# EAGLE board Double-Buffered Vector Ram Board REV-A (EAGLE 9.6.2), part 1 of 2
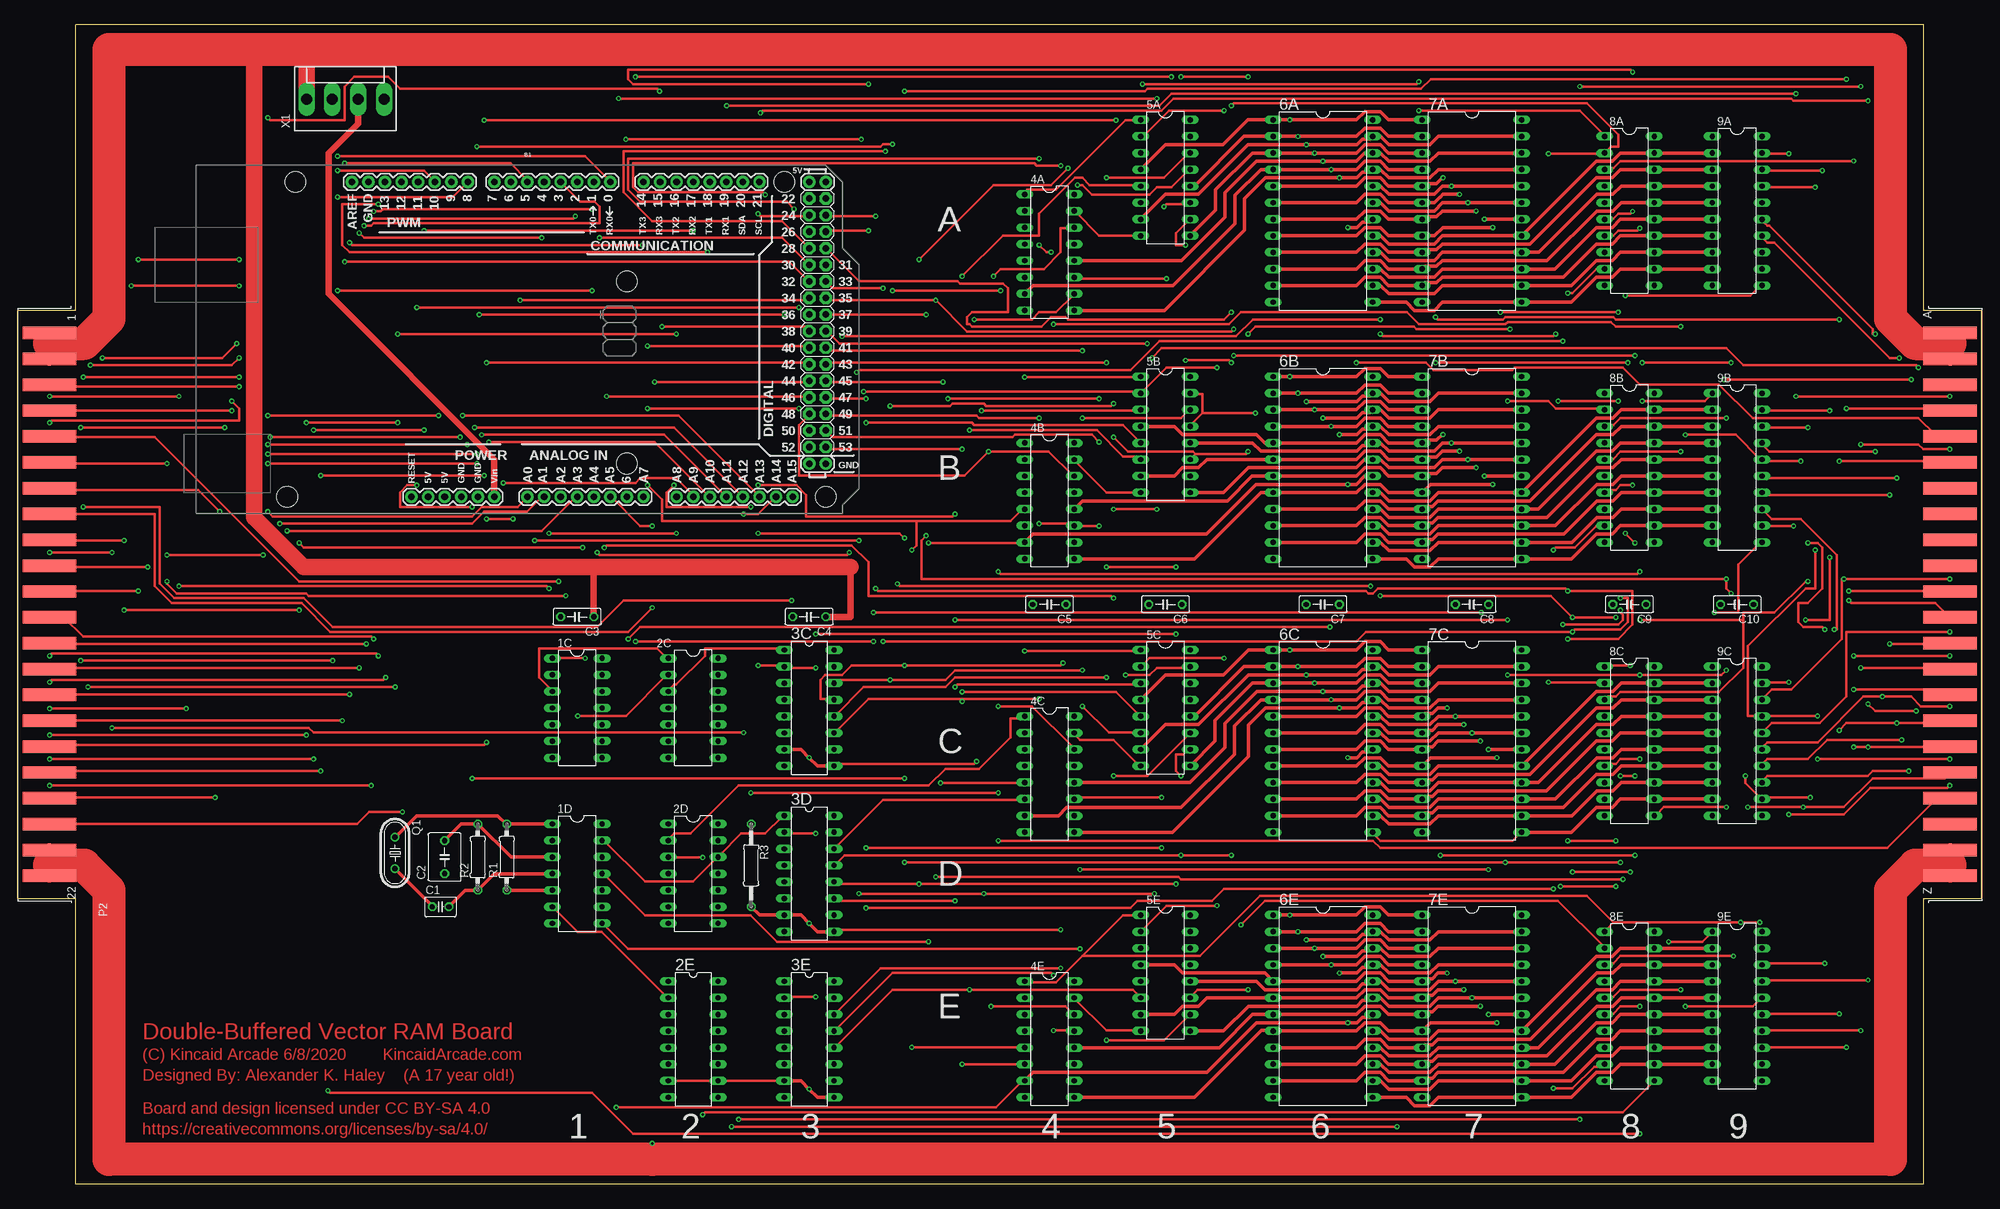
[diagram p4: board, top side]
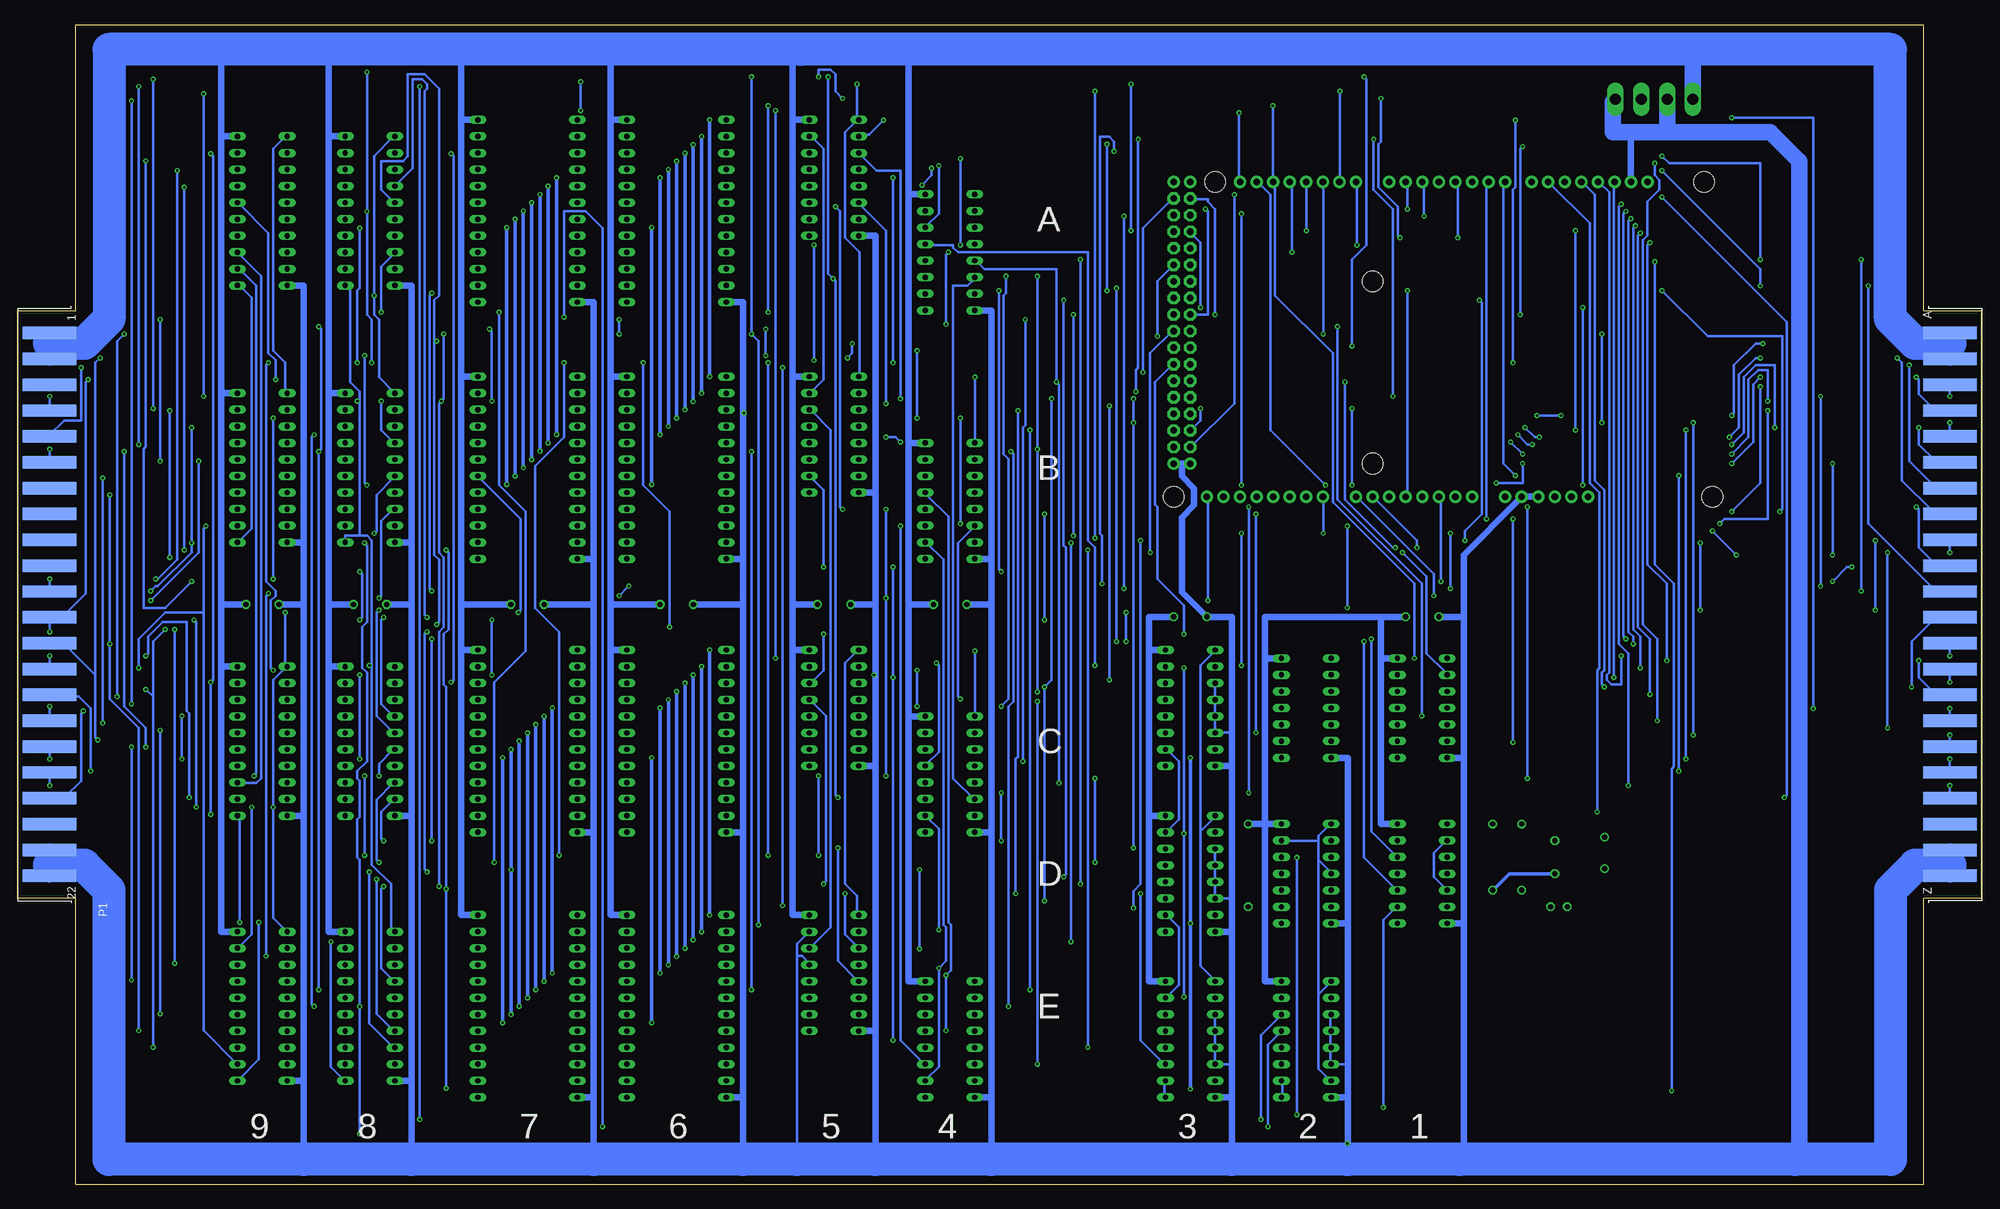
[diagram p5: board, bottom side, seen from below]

Size 300.99 x 177.8 mm. Coordinates in mm from the lower left corner, seen from the top.
Outline: 292.1,0 292.1,43.81 300.99,43.81 300.99,133.99 292.1,133.99 292.1,177.8 291.46,177.8 8.89,177.8 8.89,176.53 8.89,133.99 0,133.99 0,43.81 8.89,43.81 8.89,0 292.1,0
Copper layers (1*16): Top 0.035mm / dielectric 1.5mm / Bottom 0.035mm
Design rules "default": minimum track width 6mil, minimum drill 0.35mm, track to track 6mil, track to pad 6mil, pad to pad 6mil, via to via 6mil, smd to smd 6mil, copper to edge 40mil, drill to drill 6mil, minimum pad ring 10mil, minimum via ring 8mil, stop-mask expansion 4mil, vias tented up to drill 0mil, thermal gap 10mil
Net classes: 0 default: width 0.381 mm, clearance 0.356 mm

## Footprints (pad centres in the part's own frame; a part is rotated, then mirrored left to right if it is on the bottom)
DIL14 = drill 0.813 long: 1 -7.62,-3.81; 2 -5.08,-3.81; 3 -2.54,-3.81; 4 0,-3.81; 5 2.54,-3.81; 6 5.08,-3.81; 7 7.62,-3.81; 8 7.62,3.81; 9 5.08,3.81; 10 2.54,3.81; 11 0,3.81; 12 -2.54,3.81; 13 -5.08,3.81; 14 -7.62,3.81
DIL16 = drill 0.813 long: 1 -8.89,-3.81; 2 -6.35,-3.81; 3 -3.81,-3.81; 4 -1.27,-3.81; 5 1.27,-3.81; 6 3.81,-3.81; 7 6.35,-3.81; 8 8.89,-3.81; 9 8.89,3.81; 10 6.35,3.81; 11 3.81,3.81; 12 1.27,3.81; 13 -1.27,3.81; 14 -3.81,3.81; 15 -6.35,3.81; 16 -8.89,3.81
DIL24 = drill 0.813 long: 1 -13.97,-7.62; 2 -11.43,-7.62; 3 -8.89,-7.62; 4 -6.35,-7.62; 5 -3.81,-7.62; 6 -1.27,-7.62; 7 1.27,-7.62; 8 3.81,-7.62; 9 6.35,-7.62; 10 8.89,-7.62; 11 11.43,-7.62; 12 13.97,-7.62; 13 13.97,7.62; 14 11.43,7.62; 15 8.89,7.62; 16 6.35,7.62; 17 3.81,7.62; 18 1.27,7.62; 19 -1.27,7.62; 20 -3.81,7.62; 21 -6.35,7.62; 22 -8.89,7.62; 23 -11.43,7.62; 24 -13.97,7.62
DIL20 = drill 0.813 long: 1 -11.43,-3.81; 2 -8.89,-3.81; 3 -6.35,-3.81; 4 -3.81,-3.81; 5 -1.27,-3.81; 6 1.27,-3.81; 7 3.81,-3.81; 8 6.35,-3.81; 9 8.89,-3.81; 10 11.43,-3.81; 11 11.43,3.81; 12 8.89,3.81; 13 6.35,3.81; 14 3.81,3.81; 15 1.27,3.81; 16 -1.27,3.81; 17 -3.81,3.81; 18 -6.35,3.81; 19 -8.89,3.81; 20 -11.43,3.81
ARDUINO_MEGA = drill 1.016 pad 1.88: 0 13.97,24.13; 1 11.43,24.13; 2 8.89,24.13; 3 6.35,24.13; 3.3V -13.97,-24.13; 4 3.81,24.13; 5 1.27,24.13; 5V@0 -11.43,-24.13; 5V@1 44.45,24.13; 5V@2 46.99,24.13; 6 -1.27,24.13; 7 -3.81,24.13; 8 -7.874,24.13; 9 -10.414,24.13; 10 -12.954,24.13; 11 -15.494,24.13; 12 -18.034,24.13; 13 -20.574,24.13; 14 19.05,24.13; 15 21.59,24.13; 16 24.13,24.13; 17 26.67,24.13; 18 29.21,24.13; 19 31.75,24.13; 20 34.29,24.13; 21 36.83,24.13; A0 1.27,-24.13; A1 3.81,-24.13; A2 6.35,-24.13; A3 8.89,-24.13; A4 11.43,-24.13; A5 13.97,-24.13; A6 16.51,-24.13; A7 19.05,-24.13; A8 24.13,-24.13; A9 26.67,-24.13; A10 29.21,-24.13; A11 31.75,-24.13; A12 34.29,-24.13; A13 36.83,-24.13; A14 39.37,-24.13; A15 41.91,-24.13; AREF -25.654,24.13; GND@0 -8.89,-24.13; GND@1 -6.35,-24.13; GND@2 44.45,-19.05; GND@3 46.99,-19.05; GND@4 -23.114,24.13; RESET -16.51,-24.13; VIN -3.81,-24.13 | drill 1.016 pad 1.88 octagon: 22 44.45,21.59; 23 46.99,21.59; 24 44.45,19.05; 25 46.99,19.05; 26 44.45,16.51; 27 46.99,16.51; 28 44.45,13.97; 29 46.99,13.97; 30 44.45,11.43; 31 46.99,11.43; 32 44.45,8.89; 33 46.99,8.89; 34 44.45,6.35; 35 46.99,6.35; 36 44.45,3.81; 37 46.99,3.81; 38 44.45,1.27; 39 46.99,1.27; 40 44.45,-1.27; 41 46.99,-1.27; 42 44.45,-3.81; 43 46.99,-3.81; 44 44.45,-6.35; 45 46.99,-6.35; 46 44.45,-8.89; 47 46.99,-8.89; 48 44.45,-11.43; 49 46.99,-11.43; 50 44.45,-13.97; 51 46.99,-13.97; 52 44.45,-16.51; 53 46.99,-16.51 | hole 3.2: -34.29,24.13; -35.56,-24.13; 16.51,8.89; 16.51,-19.05; 40.64,24.13; 46.99,-24.13
C025-030X050 = drill 0.813 octagon: 1 -1.27,0; 2 1.27,0
C050-050X075 = drill 0.813 octagon: 1 -2.54,0; 2 2.54,0
C050-025X075 = drill 0.813 octagon: 1 -2.54,0; 2 2.54,0
44PINEDGE = smd 1.905 x 8.255: 1 -41.605,4.826; 2 -37.643,4.826; 3 -33.68,4.826; 4 -29.718,4.826; 5 -25.756,4.826; 6 -21.793,4.826; 7 -17.831,4.826; 8 -13.868,4.826; 9 -9.906,4.826; 10 -5.944,4.826; 11 -1.981,4.826; 12 1.981,4.826; 13 5.944,4.826; 14 9.906,4.826; 15 13.868,4.826; 16 17.831,4.826; 17 21.793,4.826; 18 25.756,4.826; 19 29.718,4.826; 20 33.68,4.826; 21 37.643,4.826; 22 41.605,4.826 | smd 1.905 x 8.255 bottom: A -41.605,4.826; B -37.643,4.826; C -33.68,4.826; D -29.718,4.826; E -25.756,4.826; F -21.793,4.826; H -17.831,4.826; J -13.868,4.826; K -9.906,4.826; L -5.944,4.826; M -1.981,4.826; N 1.981,4.826; P 5.944,4.826; R 9.906,4.826; S 13.868,4.826; T 17.831,4.826; U 21.793,4.826; V 25.756,4.826; W 29.718,4.826; X 33.68,4.826; Y 37.643,4.826; Z 41.605,4.826
HC49/S = drill 0.813: 1 -2.413,0; 2 2.413,0
0207/10 = drill 0.813 octagon: 1 -5.08,0; 2 5.08,0
0207/12 = drill 0.813 octagon: 1 -6.35,0; 2 6.35,0
KK-156-4 = drill 1.7 pad 2.184 long: 1 -5.94,0; 2 -1.98,0; 3 1.98,0; 4 5.94,0

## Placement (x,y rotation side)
1C  7432N  [DIL14]  85.72,73.03 270 top
1D  7404N  [DIL14]  85.72,47.62 270 top
2C  7400N  [DIL14]  103.5,73.03 270 top
2D  74107N  [DIL14]  103.5,47.62 270 top
2E  74161N  [DIL16]  103.5,22.23 270 top
3C  74161N  [DIL16]  121.28,73.03 270 top
3D  74161N  [DIL16]  121.28,47.62 270 top
3E  74161N  [DIL16]  121.28,22.23 270 top
4A  74157N  [DIL16]  158.12,142.88 270 top
4B  74157N  [DIL16]  158.12,104.78 270 top
4C  74157N  [DIL16]  158.12,62.87 270 top
4E  74157N  [DIL16]  158.12,22.23 270 top
5A  74157N  [DIL16]  175.9,154.31 270 top
5B  74157N  [DIL16]  175.9,114.94 270 top
5C  74157N  [DIL16]  175.9,73.03 270 top
5E  74157N  [DIL16]  175.9,32.38 270 top
6A  6116P-70  [DIL24]  200.03,149.22 270 top
6B  6116P-70  [DIL24]  200.03,109.86 270 top
6C  6116P-70  [DIL24]  200.03,67.94 270 top
6E  6116P-70  [DIL24]  200.03,27.3 270 top
7A  6116P-70  [DIL24]  222.88,149.22 270 top
7B  6116P-70  [DIL24]  222.88,109.86 270 top
7C  6116P-70  [DIL24]  222.88,67.94 270 top
7E  6116P-70  [DIL24]  222.88,27.3 270 top
8A  74HC573N  [DIL20]  247.01,149.22 270 top
8B  74HC573N  [DIL20]  247.01,109.86 270 top
8C  74HC573N  [DIL20]  247.01,67.94 270 top
8E  74HC573N  [DIL20]  247.01,27.3 270 top
9A  74HC573N  [DIL20]  263.52,149.22 270 top
9B  74HC573N  [DIL20]  263.52,109.86 270 top
9C  74HC573N  [DIL20]  263.52,67.94 270 top
9E  74HC573N  [DIL20]  263.52,27.3 270 top
B1  ARDUINO_MEGA_R3FULL  [ARDUINO_MEGA]  76.83,129.54 0 top
C1  100pf  [C025-030X050]  64.77,42.55 0 top
C2  .1uf  [C050-050X075]  65.41,50.16 90 top
C3  .1uf  [C050-025X075]  85.72,87 180 top
C4  .1uf  [C050-025X075]  121.28,87 180 top
C5  .1uf  [C050-025X075]  158.12,88.9 180 top
C6  .1uf  [C050-025X075]  175.9,88.9 180 top
C7  .1uf  [C050-025X075]  200.03,88.9 180 top
C8  .1uf  [C050-025X075]  222.88,88.9 180 top
C9  .1uf  [C050-025X075]  247.01,88.9 180 top
C10  .1uf  [C050-025X075]  263.52,88.9 180 top
P1  44PINEDGE  [44PINEDGE]  300.99,88.9 270 bottom
P2  44PINEDGE  [44PINEDGE]  0,88.9 270 top
Q1  10MHZ  [HC49/S]  57.78,50.8 270 top
R1  330  [0207/10]  74.93,50.16 90 top
R2  330  [0207/10]  70.48,50.16 90 top
R3  1K  [0207/12]  112.39,48.9 270 top
X1  [KK-156-4]  50.16,166.37 0 top

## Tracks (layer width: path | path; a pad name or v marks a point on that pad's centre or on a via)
2.5MHZ  (via drill 0.35)
  Top 0.381: v211.4,8.84 v109.39,8.84 | v217.3,132.96 217.66,132.59 227.61,132.59 227.98,132.96 244.55,132.96 244.92,132.59 v279.17,132.59 | v279.17,110.86 296.11,110.86 P1.F
  Bottom 0.381: v109.39,8.84 109.39,21.36 107.54,23.2 2E.13 | v211.4,8.84 211.4,146.58 213.98,149.16 217.3,149.16 v217.3,132.96 | v279.17,110.86 v279.17,132.59
5MHZ  (via drill 0.35)
  Top 0.381: v239.4,9.94 v110.49,9.94 | v282.49,168.31 v239.4,168.31 | v282.49,113.44 291.32,113.44 292.06,112.7 v296.11,112.7
  Bottom 0.381: v110.49,9.94 110.49,22.84 107.54,25.78 2E.14 | v239.4,168.31 v239.4,9.94 | v282.49,113.44 v282.49,168.31 | v296.11,112.7 296.11,110.86 P1.6
10MHZ
  Top 0.381: 2E.2 99.44,28.73 89.5,38.67 85.81,38.67 82.13,42.35 1D.6
+12VDC
  Top 1.016: X1.3 52.15,162.63 47.62,158.12 47.62,136.53 73.03,111.12 B1.VIN
/CS_A  (via drill 0.35)
  Top 0.381: v131.12,83.24 v94.65,83.24 | v224.29,87.66 v131.12,87.66
  Top 0.508: 7A.18 v224.79,147.96 | 7B.18 v224.79,108.58
  Bottom 0.381: v94.65,83.24 94.65,50.09 89.86,45.3 1D.10 | v131.12,87.66 v131.12,83.24 | v224.29,87.66 223.93,88.02 223.93,102.02 230.19,108.28 7B.18
  Bottom 0.508: v224.79,108.58 v224.79,147.96
/CS_B  (via drill 0.35)
  Top 0.381: v162.79,36.09 93.55,36.09 89.86,39.78 1D.8 | v225.4,48.25 v162.79,48.25
  Top 0.508: 7C.18 v225.43,66.67 | 7E.18 v225.43,26.04
  Bottom 0.381: v162.79,48.25 v162.79,36.09 | v225.4,48.25 225.43,48.25
  Bottom 0.508: v225.43,26.04 225.43,48.25 v225.43,66.67
/RESETVRAMPC
  Top 0.381: 2C.3 99.81,75.87 100.55,76.61 100.91,76.61 105.33,81.03 105.33,82.13 117.12,82.13 3C.1 | 3D.1 117.12,56.35 114.54,53.77 110.86,53.77 107.54,50.46 2D.12 107.17,50.09 103.49,46.41 96.13,46.41 89.86,52.67 1D.13
  Bottom 0.381: 119.7,54.14 119.7,33.52 117.49,31.3 3E.1 | 119.7,54.14 117.49,56.35 3D.1 | 119.7,54.14 119.7,79.55 117.49,81.76 3C.1
/TTLINVX  (via drill 0.35)
  Top 0.381: v100.55,107.17 99.44,106.07 99.44,103.86 v112.33,103.86 | v150.27,60.03 v112.33,60.03 | v150.27,52.67 207.72,52.67 208.83,51.56 286.54,51.56 293.9,58.93 296.11,58.93 P1.W
  Bottom 0.381: v100.55,107.17 109.02,115.65 109.02,151.74 110.86,153.58 B1.20 | v112.33,60.03 v112.33,103.86 | v150.27,52.67 v150.27,60.03
/TTLINVY  (via drill 0.35)
  Top 0.381: v113.81,164.26 114.17,164.63 175.31,164.63 177.15,166.47 271.81,166.47 272.17,166.1 v283.59,166.1 | v283.59,73.66 284.7,72.56 v290.96,72.56
  Bottom 0.381: v113.81,164.26 113.81,153.95 B1.21 | v283.59,73.66 v283.59,166.1 | v290.96,72.56 291.32,72.19 291.32,61.87 293.9,59.3 296.11,59.3 P1.19
/VRAMBANKSELECT  (via drill 0.35)
  Top 0.381: 163.16,34.99 169.42,41.25 172,41.25 5E.1 | 163.16,34.99 159.11,30.94 154.32,30.94 4E.1 | 2D.2 99.81,53.03 100.55,53.77 103.12,53.77 110.49,61.14 139.59,61.14 142.16,63.72 147.32,63.72 152.11,68.5 152.11,71.45 153.95,71.45 4C.1 | v154.32,81.76 172,81.76 5C.1 | 244.55,40.15 243.45,39.04 8E.1 | v267.02,40.15 v264.07,40.15 244.55,40.15 | v247.13,79.55 243.45,79.55 8C.1 | v248.97,120.07 258.55,120.07 259.65,121.17 9B.1 | 163.16,34.99 181.2,34.99 190.41,44.2 240.5,44.2 244.55,40.15
  Bottom 0.381: 5C.1 172.36,81.76 174.21,79.92 174.21,46.04 172.36,44.2 172.36,41.62 5E.1 | v154.32,81.76 154.32,71.82 4C.1 | v267.02,40.15 267.02,56.35 9C.11 | v264.07,40.15 264.07,19.15 267.02,16.2 9E.11 | 246.76,79.92 v247.13,79.55 | 246.76,79.92 246.76,98.7 247.5,99.44 248.6,99.44 | 248.6,99.44 250.81,99.44 250.81,98.7 8B.11 | 248.6,99.44 248.6,120.07 | 248.6,120.07 248.6,121.54 250.08,123.01 250.08,137.01 250.81,137.74 8A.11 | 248.6,120.07 v248.97,120.07 | 9A.1 260.02,160.58 261.86,158.74 261.86,127.8 260.02,125.96 260.02,121.54 9B.1 | 246.76,79.92 246.76,48.98 243.81,46.04 243.81,39.41 243.45,39.04 8E.1
A0_A  (via drill 0.35)
  Top 0.508: 6A.8 205.19,145.41 206.46,146.69 208.83,146.69 210.1,145.41 7A.8 217.13,145.41 218.41,146.69 v226.06,146.69 | v226.06,107.31 216.53,107.31 7B.8 210.1,106.05 208.83,107.31 206.46,107.31 205.19,106.05 6B.8 190.5,106.05 180.34,95.89 4B.9
  Bottom 0.508: v226.06,146.69 v226.06,107.31
A0_B  (via drill 0.35)
  Top 0.508: 6C.8 205.19,64.14 206.46,65.41 208.83,65.41 210.1,64.14 7C.8 216.53,65.41 v226.69,65.41 | v226.69,24.77 216.53,24.77 7E.8 210.1,23.5 208.83,24.77 206.46,24.77 205.19,23.5 6E.8 192.33,23.57 190.58,23.57 180.34,13.34 4E.9
  Bottom 0.508: v226.69,65.41 v226.69,24.77
A1_A  (via drill 0.35)
  Top 0.508: 6A.7 205.19,147.96 206.46,149.22 208.83,149.22 210.1,147.96 7A.7 215.67,148.36 217.44,148.36 218.31,149.22 v223.52,149.22 | v223.52,109.86 218.31,109.86 217.44,108.99 215.67,108.99 7B.7 210.1,108.58 208.83,109.86 206.46,109.86 205.19,108.58 6B.7 189.18,108.58 185.37,104.78 163.19,104.78 4B.12
  Bottom 0.508: v223.52,149.22 v223.52,109.86
A1_B  (via drill 0.35)
  Top 0.508: 6C.7 205.19,66.67 206.46,67.94 208.83,67.94 210.1,66.67 7C.7 215.67,67.08 216.81,67.08 217.67,67.94 v224.16,67.94 | v224.16,27.3 217.67,27.3 216.81,26.44 215.67,26.44 7E.7 210.1,26.04 208.83,27.3 206.46,27.3 205.19,26.04 6E.7 189.23,26.04 184.15,20.95 4E.12
  Bottom 0.508: v224.16,67.94 v224.16,27.3
A2_A  (via drill 0.35)
  Top 0.508: 6A.6 205.19,150.5 206.46,151.76 208.83,151.76 210.1,150.5 7A.6 217.13,150.5 218,151.36 218.03,151.36 218.44,151.76 v220.98,151.76 | v220.98,112.39 218.31,112.39 217.44,111.53 215.67,111.53 7B.6 210.1,111.12 208.83,112.39 206.46,112.39 205.19,111.12 6B.6 182.25,111.12 180.97,109.86 178.52,109.86 177.25,108.58 5B.7
  Bottom 0.508: v220.98,151.76 v220.98,112.39
A2_B  (via drill 0.35)
  Top 0.508: 6C.6 205.19,69.22 206.46,70.48 208.83,70.48 210.1,69.22 7C.6 215.67,69.62 216.81,69.62 217.67,70.48 v221.62,70.48 | v221.62,29.84 217.67,29.84 216.81,28.98 215.67,28.98 7E.6 210.1,28.57 208.83,29.84 206.46,29.84 205.19,28.57 6E.6 182.25,28.57 180.97,27.3 178.52,27.3 177.25,26.04 5E.7
  Bottom 0.508: v221.62,70.48 v221.62,29.84
A3_A  (via drill 0.35)
  Top 0.508: 6A.5 205.19,153.03 206.46,154.31 208.83,154.31 210.1,153.03 7A.5 215.67,153.44 217.44,153.44 218.31,154.31 v218.44,154.31 | v218.44,114.94 218.31,114.94 217.44,114.07 215.67,114.07 7B.5 210.1,113.67 208.83,114.94 206.46,114.94 205.19,113.67 6B.5 191.13,113.67 189.87,114.94 178.52,114.94 177.25,116.2 5B.4
  Bottom 0.508: v218.44,154.31 v218.44,114.94
A3_B  (via drill 0.35)
  Top 0.508: 6C.5 205.19,71.75 206.46,73.03 208.83,73.03 210.1,71.75 7C.5 215.67,72.16 216.81,72.16 217.67,73.03 v219.07,73.03 | v219.07,32.38 217.67,32.38 216.81,31.52 215.67,31.52 7E.5 210.1,31.11 208.83,32.38 206.46,32.38 205.19,31.11 6E.5 191.13,32.38 178.52,32.38 177.25,33.66 5E.4
  Bottom 0.508: v219.07,73.03 v219.07,32.38
A4_A  (via drill 0.35)
  Top 0.508: 7A.4 210.1,155.57 208.83,156.84 206.46,156.84 205.19,155.57 v201.29,155.57 6A.4 190.5,155.57 186.54,151.61 186.54,147.3 177.03,137.79 155.57,137.79 4A.7 | 6B.4 v201.29,116.2 205.19,116.2 206.46,117.47 208.83,117.47 210.1,116.2 7B.4
  Bottom 0.508: v201.29,155.57 v201.29,116.2
A4_B  (via drill 0.35)
  Top 0.508: 7C.4 210.1,74.3 208.83,75.56 206.46,75.56 205.19,74.3 v201.29,74.3 6C.4 190.5,74.3 186.46,70.26 186.46,65.94 178.3,57.78 160.74,57.78 159.47,56.52 4C.7 | 6E.4 v201.29,33.66 205.19,33.66 206.46,34.92 208.83,34.92 210.1,33.66 7E.4
  Bottom 0.508: v201.29,74.3 v201.29,33.66
A5_A  (via drill 0.35)
  Top 0.508: 7A.3 210.1,158.12 208.83,159.38 206.46,159.38 205.19,158.12 v198.75,158.12 6A.3 189.19,158.12 183.54,152.46 183.54,149.33 179.71,145.5 5A.9 | 6B.3 v198.75,118.75 205.19,118.75 206.46,120.02 208.83,120.02 210.1,118.75 7B.3
  Bottom 0.508: v198.75,158.12 v198.75,118.75
A5_B  (via drill 0.35)
  Top 0.508: 7C.3 210.1,76.83 208.83,78.11 206.46,78.11 205.19,76.83 v198.75,76.83 6C.3 189.23,76.83 183.51,71.12 183.51,67.94 5C.9 | 6E.3 v198.75,36.2 205.19,36.2 206.46,37.47 208.83,37.47 210.1,36.2 7E.3
  Bottom 0.508: v198.75,76.83 v198.75,36.2
A6_A  (via drill 0.35)
  Top 0.508: 7A.2 210.1,160.66 208.83,161.93 206.46,161.93 205.19,160.66 v196.22,160.66 6A.2 187.96,160.66 180.34,153.03 5A.12 | 6B.2 v196.22,121.28 205.19,121.28 206.46,122.56 208.83,122.56 210.1,121.28 7B.2
  Bottom 0.508: v196.22,160.66 v196.22,121.28
A6_B  (via drill 0.35)
  Top 0.508: 7C.2 210.1,79.38 208.83,80.64 206.46,80.64 205.19,79.38 v196.22,79.38 6C.2 187.96,79.38 180.34,71.75 5C.12 | 6E.2 v196.22,38.73 205.19,38.73 206.46,40.01 208.83,40.01 210.1,38.73 7E.2
  Bottom 0.508: v196.22,79.38 v196.22,38.73
A7_A  (via drill 0.35)
  Top 0.508: 7A.1 210.1,163.19 208.83,164.47 206.46,164.47 205.19,163.19 v194.94,163.19 6A.1 188.51,163.19 184.7,159.38 175.9,159.38 5A.4 | 6B.1 v194.94,123.83 205.19,123.83 206.46,125.09 208.83,125.09 210.1,123.83 7B.1
  Bottom 0.508: v194.94,123.83 v194.94,163.19
A7_B  (via drill 0.35)
  Top 0.508: 7C.1 210.1,81.92 208.83,83.19 206.46,83.19 205.19,81.92 v194.94,81.92 6C.1 188.59,81.92 184.78,78.11 175.9,78.11 5C.4 | 6E.1 v194.94,41.27 205.19,41.27 206.46,42.55 208.83,42.55 210.1,41.27 7E.1
  Bottom 0.508: v194.94,41.27 v194.94,81.92
A8_A  (via drill 0.35)
  Top 0.508: 7B.23 217.72,121.28 216.45,120.02 210.15,120.02 208.88,121.28 6B.23 207.24,120.88 206.1,120.88 205.24,120.02 v197.49,120.02 | 7A.23 217.72,160.66 216.45,159.38 210.15,159.38 208.88,160.66 6A.23 207.24,160.25 206.1,160.25 205.24,159.38 v197.49,159.38 188.56,159.38 180.94,151.76 175.9,151.76 5A.7
  Bottom 0.508: v197.49,120.02 v197.49,159.38
A8_B  (via drill 0.35)
  Top 0.508: 7C.23 217.72,79.38 216.45,78.11 210.15,78.11 208.88,79.38 6C.23 207.24,78.97 206.1,78.97 205.24,78.11 v197.49,78.11 188.59,78.11 180.97,70.48 175.9,70.48 5C.7 | 7E.23 217.72,38.73 216.45,37.47 210.15,37.47 208.88,38.73 6E.23 207.24,38.33 206.1,38.33 205.24,37.47 v197.49,37.47
  Bottom 0.508: v197.49,37.47 v197.49,78.11
A9_A  (via drill 0.35)
  Top 0.508: 7B.22 217.72,118.75 216.45,117.47 210.15,117.47 208.88,118.75 6B.22 207.24,118.34 206.1,118.34 205.24,117.47 v200.03,117.47 | 7A.22 217.72,158.12 216.45,156.84 210.15,156.84 208.88,158.12 6A.22 206.41,158.12 205.14,156.84 v200.03,156.84 189.87,156.84 185.04,152.02 185.04,148.29 178.35,141.6 4A.12
  Bottom 0.508: v200.03,117.47 v200.03,156.84
A9_B  (via drill 0.35)
  Top 0.508: 7C.22 217.72,76.83 216.45,75.56 210.15,75.56 208.88,76.83 6C.22 207.24,76.43 206.1,76.43 205.24,75.56 v200.03,75.56 189.95,75.56 185.01,70.63 185.01,66.99 179.62,61.59 4C.12 | 7E.22 217.72,36.2 216.45,34.92 210.15,34.92 208.88,36.2 6E.22 207.24,35.79 206.1,35.79 205.24,34.92 v200.03,34.92
  Bottom 0.508: v200.03,34.92 v200.03,75.56
A10_A  (via drill 0.35)
  Top 0.508: 7B.19 v222.25,111.12 218.36,111.12 217.09,109.86 210.15,109.86 208.88,111.12 6B.19 206.41,111.12 205.14,109.86 188.59,109.86 184.78,106.05 5B.9 | 6A.19 208.88,150.5 210.15,149.22 217.09,149.22 218.36,150.5 v222.25,150.5 7A.19
  Bottom 0.508: v222.25,111.12 v222.25,150.5
A10_B  (via drill 0.35)
  Top 0.508: 6C.19 208.88,69.22 210.15,67.94 216.45,67.94 217.72,69.22 v222.88,69.22 7C.19 | 7E.19 v222.88,28.57 217.72,28.57 216.45,27.3 210.15,27.3 208.88,28.57 6E.19 207.24,28.17 206.1,28.17 205.24,27.3 188.59,27.3 184.78,23.5 5E.9
  Bottom 0.508: v222.88,28.57 v222.88,69.22
CS_A  (via drill 0.35)
  Top 0.381: v139.59,37.2 116.38,37.2 112.33,41.25 96.13,41.25 89.86,47.51 1D.11 | v139.59,98.34 153.95,98.34 4B.7
  Top 0.508: 6B.18 206.41,108.58 205.14,107.31 v203.84,107.31 189.77,107.31 182.15,99.69 155.57,99.69 4B.7 | 6A.18 207.24,147.55 206.1,147.55 205.24,146.69 v203.84,146.69
  Bottom 0.381: v139.59,98.34 v139.59,37.2
  Bottom 0.508: v203.84,146.69 v203.84,107.31
CS_B  (via drill 0.35)
  Top 0.381: v91.71,11.79 149.9,11.79 153.95,15.84 4E.7
  Top 0.508: 6C.18 207.24,66.27 206.1,66.27 205.24,65.41 v203.84,65.41 | 6E.18 207.24,25.63 206.1,25.63 205.24,24.77 v203.84,24.77 189.87,24.77 182.25,17.14 155.57,17.14 4E.7
  Bottom 0.381: v91.71,11.79 91.71,40.51 89.86,42.35 1D.9
  Bottom 0.508: v203.84,65.41 v203.84,24.77
CSIN  (via drill 0.35)
  Top 0.381: v137.01,20.99 153.95,20.99 4E.5 | v137.01,97.23 137.74,97.97 137.74,101.65 | 137.74,101.65 152.11,101.65 153.95,103.49 4B.5 | v96.5,118.96 v119.7,118.96 | v96.5,107.17 98.7,104.97 98.7,101.65 137.74,101.65
  Bottom 0.381: v137.01,97.23 v137.01,20.99 | v119.7,118.96 119.7,117.12 121.17,115.65 B1.50 | v96.5,107.17 v96.5,118.96
D0  (via drill 0.35)
  Top 0.381: v48.98,157.63 86.92,157.63 90.6,153.95 B1.0 | v18.47,90.97 4.84,90.97 P2.11 | v18.47,141.8 v33.88,141.8
  Bottom 0.381: v48.98,157.63 47.88,156.53 33.88,156.53 v33.88,141.8 | v18.47,90.97 v18.47,141.8
D1  (via drill 0.35)
  Top 0.381: v88.02,149.53 55.98,149.53 55.61,149.16 v54.51,149.16 | v54.51,83.6 54.14,83.97 9.99,83.97 7.05,86.92 P2.12
  Bottom 0.381: v88.02,149.53 88.02,153.58 B1.1 | v54.51,149.16 54.88,148.79 54.88,83.97 v54.51,83.6
D2  (via drill 0.35)
  Top 0.381: v85.45,148.43 85.08,148.06 v53.77,148.06 | v53.4,82.87 4.84,82.87 P2.13
  Bottom 0.381: v85.45,148.43 85.45,153.58 B1.2 | v53.77,148.06 54.14,147.69 54.14,84.71 53.4,83.97 v53.4,82.87
D3  (via drill 0.35)
  Top 0.381: v53.03,146.95 54.14,146.95 54.51,147.32 89.13,147.32 89.13,149.9 88.39,150.63 86.18,150.63 83.24,153.58 B1.3 | v52.3,79.18 4.84,79.18 P2.14
  Bottom 0.381: v53.03,146.95 53.4,146.58 53.4,85.08 52.3,83.97 v52.3,79.18
D4  (via drill 0.35)
  Top 0.381: v80.29,145.11 53.03,145.11 v52.3,145.85 | v50.83,75.13 4.84,75.13 P2.15
  Bottom 0.381: v80.29,145.11 80.29,153.58 B1.4 | v52.3,145.85 52.67,145.48 52.67,85.45 50.83,83.6 v50.83,75.13
D5  (via drill 0.35)
  Top 0.381: v50.09,156.53 75.5,156.53 78.08,153.95 B1.5 | v49.72,71.08 4.84,71.08 P2.16
  Bottom 0.381: v50.09,156.53 50.09,154.69 49.35,153.95 49.35,152.48 51.19,150.63 51.19,145.48 51.93,144.74 51.93,85.81 49.72,83.6 v49.72,71.08
D6  (via drill 0.35)
  Top 0.381: v71.82,102.02 v75.87,102.02 | v71.82,67.77 71.45,67.4 4.84,67.4 P2.17
  Bottom 0.381: v75.87,102.02 75.87,153.58 B1.6 | v71.82,67.77 v71.82,102.02
D7  (via drill 0.35)
  Top 0.381: v46.41,108.65 v71.45,108.65 | v46.41,63.35 4.84,63.35 P2.18
  Bottom 0.381: v71.45,108.65 73.29,110.49 73.29,153.58 B1.7 | v46.41,63.35 v46.41,108.65
D8  (via drill 0.35)
  Top 0.381: B1.8 66.66,151.37 v48.98,151.37 | v30.2,59.3 4.84,59.3 P2.19
  Bottom 0.381: v48.98,151.37 29.83,132.22 29.83,59.66 v30.2,59.3
D9  (via drill 0.35)
  Top 0.381: v58.93,57.09 53.85,57.09 52.01,55.24 4.84,55.24 P2.20
  Bottom 0.381: v58.93,57.09 58.93,78.82 58.56,79.18 58.56,106.07 60.03,107.54 60.03,147.32 66.29,153.58 B1.9
D10  (via drill 0.35)
  Top 0.381: v48.98,155.42 62.24,155.42 63.72,153.95 B1.10 | v33.88,137.74 v17.36,137.74
  Bottom 0.381: v48.98,155.42 33.88,140.32 v33.88,137.74 | v17.36,137.74 17.36,101.28 7.05,90.97 4.84,90.97 P2.M
D11  (via drill 0.35)
  Top 0.381: v57.82,76.24 v10.73,76.24
  Bottom 0.381: v57.82,76.24 58.19,76.61 58.19,78.45 57.82,78.82 57.82,106.44 59.3,107.91 59.3,151.74 61.14,153.58 B1.11 | v10.73,76.24 10.73,83.24 7.05,86.92 P2.N
D12  (via drill 0.35)
  Top 0.381: v55.24,81.03 54.88,81.39 5.21,81.39 v4.84,81.03
  Bottom 0.381: v55.24,81.03 55.24,76.61 56.72,76.61 57.45,77.34 57.45,78.08 57.09,78.45 57.09,152.11 58.56,153.58 B1.12 | v4.84,81.03 4.84,82.87 P2.P
D13  (via drill 0.35)
  Top 0.381: v56.35,77.71 55.98,77.34 5.21,77.34 v4.84,76.97
  Bottom 0.381: v56.35,77.71 56.35,153.58 B1.13 | v4.84,76.97 4.84,78.82 P2.R
D14  (via drill 0.35)
  Top 0.381: v95.76,144 51.19,144 v50.83,144.37 | v9.63,80.29 v48.25,80.29
  Bottom 0.381: v95.76,144 95.76,153.58 B1.14 | v50.83,144.37 51.19,144 51.19,95.02 48.25,92.08 v48.25,80.29 | v9.63,80.29 9.63,77.71 7.05,75.13 4.84,75.13 P2.S
D15  (via drill 0.35)
  Top 0.381: v98.34,167.58 97.97,167.94 58.56,167.94 56.72,169.79 51.56,169.79 50.09,168.31 50.09,163.16 38.67,163.16 v38.3,163.53 | v4.84,72.92 v25.78,72.92
  Bottom 0.381: v98.34,167.58 98.34,153.95 B1.15 | v38.3,163.53 25.78,163.53 v25.78,72.92 | v4.84,72.92 4.84,71.08 P2.T
D16  (via drill 0.35)
  Top 0.381: v58.19,130.38 v100.91,130.38 | v44.2,116.75 v58.19,116.75 | v44.2,68.87 v4.84,68.87
  Bottom 0.381: v100.91,130.38 100.91,153.58 B1.16 | v58.19,116.75 v58.19,130.38 | v44.2,68.87 v44.2,116.75 | v4.84,68.87 4.84,67.4 P2.U
D17  (via drill 0.35)
  Top 0.381: v62.24,146.22 v103.49,146.22 | v45.3,115.65 v62.24,115.65 | v4.84,65.19 v45.3,65.19
  Bottom 0.381: v103.49,146.22 103.49,153.58 B1.17 | v62.24,115.65 v62.24,146.22 | v45.3,65.19 v45.3,115.65 | v4.84,65.19 4.84,63.35 P2.V
D18  (via drill 0.35)
  Top 0.381: v105.7,142.9 50.83,142.9 49.72,144 49.72,150.27 v55.24,150.27 | v54.14,61.14 v4.84,61.14
  Bottom 0.381: v105.7,142.9 105.7,153.58 B1.18 | v55.24,150.27 55.61,149.9 55.61,82.87 54.14,81.39 v54.14,61.14 | v4.84,61.14 4.84,59.3 P2.W
FRAMECOMPLETE  (via drill 0.35)
  Top 0.381: v86.92,80.66 82.13,80.66 1C.1 | v272.54,120.8 v296.11,120.8 | v272.54,167.21 176.78,167.21 174.94,165.37 v108.65,165.37
  Bottom 0.381: v86.92,80.66 86.92,92.08 99.44,104.6 99.44,127.43 108.28,136.27 108.28,153.58 B1.19 108.65,153.95 v108.65,165.37 | v296.11,120.8 296.11,118.96 P1.4 | v272.54,167.21 v272.54,120.8
GND  (via drill 0.35)
  Top 0.381: 181.57,118.22 179.73,116.38 5B.13 | 181.57,118.22 181.57,121.17 179.73,121.17 5B.15 | 4E.15 162.05,28.36 166.84,23.57 172,23.57 5E.8 | 4C.15 162.05,68.87 162.79,68.14 167.94,68.14 171.63,64.45 172,64.45 5C.8 | 4B.15 162.05,110.86 166.84,106.07 172,106.07 5B.8 | 4A.15 162.05,149.16 165.74,145.48 172,145.48 5A.8 | v169.79,78.08 173.47,78.08 174.57,79.18 179.36,79.18 5C.15 | v189.67,118.22 181.57,118.22 | v97.23,6.26 97.23,3.81
  Top 2.032: P2.22 4.83,48.9 P2.21 | P1.Z 296.16,48.9 P1.Y
  Top 5.08: 4.83,48.9 10.16,48.9 13.97,45.09 13.97,3.81 97.23,3.81 287.02,3.81 287.02,45.09 290.83,48.9 296.16,48.9
  Bottom 0.381: 5A.15 179.36,160.58 177.52,158.74 177.52,123.38 179.36,121.54 5B.15 | 3C.3 117.49,76.61 117.49,74.4 3C.4 117.49,74.03 117.49,71.82 3C.5 117.49,71.45 117.49,69.24 3C.6 117.12,69.24 114.94,69.24 | 3D.3 117.49,51.19 117.49,48.98 3D.4 117.49,48.62 117.49,46.41 3D.5 117.49,46.04 117.49,43.83 3D.6 117.12,43.83 114.94,43.83 | 3E.3 117.49,25.78 117.49,23.57 3E.4 117.49,23.2 117.49,20.99 3E.5 117.49,20.62 117.49,18.41 3E.6 114.94,18.41 | 2E.3 99.81,25.78 99.81,23.57 2E.4 99.81,23.2 99.81,20.99 2E.5 99.81,20.62 99.81,18.41 2E.6 97.16,18.41 | 181.57,34.99 180.84,34.99 179.73,33.88 5E.13 | 181.57,34.99 181.57,36.83 179.73,38.67 5E.15 | v169.79,78.08 169.54,78.08 | 181.57,3.81 181.57,34.99 | v189.67,118.22 189.87,118.22 | v97.23,6.26 97.23,3.81
  Bottom 1.016: 4E.8 151.76,13.34 | 151.76,13.34 151.76,3.81 | 6E.12 189.87,13.34 | 189.87,3.81 189.87,13.34 | 5E.8 169.54,23.5 | 169.54,3.81 169.54,23.5 | 7E.12 212.72,13.34 | 212.72,3.81 212.72,13.34 | 8E.10 240.66,15.88 | 240.66,3.81 240.66,15.88 | 9E.10 257.18,15.88 | 257.18,15.88 257.18,3.81 | 257.18,15.88 257.18,56.52 | 257.18,56.52 257.18,88.9 | 257.18,88.9 257.18,98.42 | 257.18,98.42 257.18,137.79 9A.10 | 257.18,98.42 9B.10 | 257.18,88.9 C10.2 | 257.18,56.52 9C.10 | 240.66,15.88 240.66,56.52 | 240.66,56.52 240.66,88.9 | 240.66,88.9 240.66,98.42 | 240.66,98.42 240.66,137.79 8A.10 | 240.66,98.42 8B.10 | 8C.10 240.66,56.52 | 212.72,13.34 212.72,53.98 | 212.72,53.98 212.72,88.9 | 212.72,88.9 212.72,95.89 | 212.72,95.89 212.72,135.25 7A.12 | 212.72,95.89 7B.12 | 212.72,53.98 7C.12 | 189.87,13.34 189.87,53.98 | 189.87,53.98 189.87,88.9 | 189.87,88.9 189.87,95.89 | 189.87,95.89 189.87,118.22 189.87,135.25 6A.12 | 189.87,95.89 6B.12 | 189.87,53.98 6C.12 | 169.54,23.5 169.54,64.14 | 169.54,64.14 169.54,78.08 169.54,88.9 | 169.54,88.9 169.54,106.05 | 169.54,106.05 169.54,145.41 5A.8 | 169.54,106.05 5B.8 | 169.54,64.14 5C.8 | 151.76,13.34 151.76,53.98 | 151.76,53.98 151.76,88.9 | 151.76,88.9 151.76,95.89 | 151.76,95.89 151.76,133.99 4A.8 | 151.76,95.89 4B.8 | 151.76,53.98 4C.8 | 240.66,88.9 C9.2 | C8.2 212.72,88.9 | C7.2 189.87,88.9 | C6.2 169.54,88.9 | C5.2 151.76,88.9 | 3E.8 114.94,13.34 | 114.94,13.34 114.94,3.81 | 114.94,13.34 114.94,18.41 114.94,38.73 | 114.94,38.73 114.94,43.83 114.94,64.14 | 3C.8 114.94,64.14 | 114.94,38.73 3D.8 | 2E.8 97.16,13.34 | 97.16,13.34 97.16,3.81 | 97.16,13.34 97.16,18.41 97.16,40.01 | 97.16,40.01 97.16,65.41 2C.7 | 2D.7 97.16,40.01 | 114.94,64.14 114.94,69.24 114.94,87 C4.2 122.56,90.81 122.56,102.26 120.7,104.12 120.7,106.7 122.56,108.56 122.56,110.49
  Bottom 1.016: 1D.7 79.38,40.01 | 79.38,40.01 79.38,4.45 80.01,3.81 | 79.38,40.01 79.38,65.41 | 79.38,65.41 1C.7 | 79.38,65.41 79.38,87 | 79.38,87 C3.2 | B1.GND@4 53.72,161.04 53.98,161.29 | 122.56,110.49 B1.GND@2 | 122.56,110.49 B1.GND@3 | B1.GND@0 B1.GND@1 71.22,104.67 71.22,104.66 79.38,96.51 79.38,87
  Bottom 2.032: P2.22 4.83,48.9 P2.21 | P1.Z 296.16,48.9 P1.Y
  Bottom 2.54: X1.2 48.19,161.37 48.26,161.29 | 48.26,161.29 53.98,161.29 56.52,161.29 56.52,165.96 X1.4 | 48.26,161.29 32.38,161.29 27.94,156.84 27.94,4.45 28.57,3.81
  Bottom 5.08: 4.83,48.9 10.16,48.9 13.97,45.09 13.97,3.81 28.57,3.81 80.01,3.81 97.16,3.81 97.23,3.81 114.94,3.81 151.76,3.81 169.54,3.81 181.57,3.81 189.87,3.81 212.72,3.81 240.66,3.81 257.18,3.81 287.02,3.81 287.02,45.09 290.83,48.9 296.16,48.9
N$2
  Top 0.381: 1C.3 81.76,75.87 79.92,77.71 79.92,82.13 97.97,82.13 99.44,80.66 2C.1
N$5
  Bottom 0.381: 3D.15 124.85,54.14 123.01,55.98 123.01,64.82 124.85,66.66 3C.10
N$6
  Bottom 0.381: 3E.15 124.85,28.73 123.01,30.57 123.01,39.41 124.85,41.25 3D.10
N$48
  Top 0.508: 1D.1 R1.2 74.82,55.24 73.55,56.52 61.09,56.52 Q1.1
N$52
  Top 0.508: 1D.5 R1.1
  Bottom 0.381: 1D.5 83.97,47.14 83.97,50.83 82.13,52.67 1D.2
  Bottom 0.508: C2.1 72.39,47.62 R1.1
N$61
  Top 0.508: 1D.3 75.56,50.16 R2.2 67.94,55.24 C2.2
N$69
  Top 0.508: Q1.2 63.5,42.67 C1.1
N$74
  Top 0.508: 1D.4 73.03,47.62 R2.1 68.58,45.09 C1.2
OE_A  (via drill 0.35)
  Top 0.508: 7B.20 v219.71,113.67 218.36,113.67 217.09,112.39 210.15,112.39 208.88,113.67 6B.20 207.24,113.26 206.1,113.26 205.24,112.39 190.5,112.39 189.23,113.67 5B.12 | 6A.20 208.88,153.03 210.15,151.76 217.09,151.76 218.36,153.03 v219.71,153.03 7A.20
  Bottom 0.508: v219.71,113.67 v219.71,153.03
OE_B  (via drill 0.35)
  Top 0.508: 6C.20 208.88,71.75 210.15,70.48 216.45,70.48 217.72,71.75 v220.34,71.75 7C.20 | 7E.20 v220.34,31.11 217.72,31.11 216.45,29.84 210.15,29.84 208.88,31.11 6E.20 207.24,30.71 206.1,30.71 205.24,29.84 191.13,29.84 189.87,31.11 5E.12
  Bottom 0.508: v220.34,31.11 v220.34,71.75
OEIN  (via drill 0.35)
  Top 0.381: v163.16,127.8 124.48,127.8 124.12,128.17 B1.41 | v163.16,117.49 178.26,117.49 179.36,118.59 5B.14
  Bottom 0.381: 5E.14 179.36,36.46 176.42,39.41 176.42,115.65 179.36,118.59 5B.14 | v163.16,117.49 v163.16,127.8
P  (via drill 0.35)
  Top 0.381: 2E.7 99.81,15.84 107.17,15.84 2E.10 107.54,15.84 117.12,15.84 3E.7 | v159.84,39.04 125.22,39.04 3D.9 | v146.58,132.59 155.42,132.59 156.53,133.69 159.11,133.69 161.68,136.27 4A.10 | v146.95,64.82 146.58,64.45 125.22,64.45 3C.9
  Top 0.508: R3.2 113.67,41.27 3D.7 120.02,41.27 v121.28,40.01 122.56,38.73 3D.9 | 3C.9 122.56,64.14 v121.28,65.41 120.02,66.67 3C.7 | 3E.9 122.56,13.34 v121.28,14.61 120.02,15.88 3E.7
  Bottom 0.381: 101.65,49.72 99.81,47.88 2D.4 | 101.65,52.67 101.65,53.4 99.81,55.24 2D.1 | 101.65,52.67 101.65,49.72 | 101.65,52.67 107.17,52.67 2D.13 | 2E.9 107.17,13.63 107.17,15.84 2E.10 | 101.65,29.1 99.81,30.94 2E.1 | 101.65,29.1 101.65,17.68 99.81,15.84 2E.7 | 101.65,29.1 101.65,49.72 | 3E.10 125.22,15.84 125.22,13.63 3E.9 | v159.84,39.04 159.84,54.51 161.68,56.35 4C.10 | v146.58,132.59 146.58,116.38 146.95,116.01 v146.95,64.82
  Bottom 0.508: v121.28,14.61 v121.28,40.01 v121.28,65.41
PORTF0  (via drill 0.35)
  Top 0.381: v38.3,103.12 39.04,102.39 69.61,102.39 71.08,103.86 76.61,103.86 78.08,105.33 B1.A0 | v33.88,122.28 4.84,122.28 P2.3
  Bottom 0.381: v38.3,103.12 33.88,107.54 v33.88,122.28
PORTF1  (via drill 0.35)
  Top 0.381: v40.15,101.28 69.61,101.28 71.45,103.12 78.08,103.12 80.29,105.33 B1.A1 | v32.78,118.59 4.84,118.59 P2.4
  Bottom 0.381: v40.15,101.28 39.41,102.02 32.78,102.02 v32.78,118.59
PORTF2  (via drill 0.35)
  Top 0.381: v82.87,92.44 43.09,92.44 20.99,114.54 4.84,114.54 P2.5
  Bottom 0.381: v82.87,92.44 82.87,105.33 B1.A2
PORTF3  (via drill 0.35)
  Top 0.381: v41.25,100.18 80.29,100.18 85.45,105.33 B1.A3 | v22.84,96.5 v37.57,96.5 | v22.84,110.49 4.84,110.49 P2.6
  Bottom 0.381: v37.57,96.5 v41.25,100.18 | v22.84,110.49 v22.84,96.5
PORTF4  (via drill 0.35)
  Top 0.381: v48.98,137.01 v88.02,137.01 | v30.94,103.12 27.62,106.44 4.84,106.44 P2.7
  Bottom 0.381: v88.02,137.01 88.02,105.7 B1.A4 | v48.98,137.01 41.99,130.01 30.57,130.01 30.57,103.49 v30.94,103.12
PORTF5  (via drill 0.35)
  Top 0.381: v97.23,100.91 95.39,100.91 90.97,105.33 B1.A5 | v97.23,88.39 93.55,84.71 47.88,84.71 43.46,89.13 23.57,89.13 20.99,91.71 20.99,102.76 4.84,102.76 P2.8
  Bottom 0.381: v97.23,88.39 v97.23,100.91
PORTF6  (via drill 0.35)
  Top 0.381: v86.55,97.6 43.83,97.6 v43.09,98.34 | v16.26,98.7 4.84,98.7 P2.9 | v16.26,88.02 v43.09,88.02
  Bottom 0.381: v86.55,97.6 86.55,98.7 93.18,105.33 B1.A6 | v43.09,88.02 v43.09,98.34 | v16.26,98.7 v16.26,88.02
PORTF7  (via drill 0.35)
  Top 0.381: v83.97,90.23 44.56,90.23 44.2,90.6 24.31,90.6 22.84,92.08 v22.84,92.44 | v19.89,94.65 4.84,94.65 P2.10
  Bottom 0.381: v83.97,90.23 83.97,93.55 95.76,105.33 B1.A7 | v22.84,92.44 20.62,94.65 v19.89,94.65
PORTK0  (via drill 0.35)
  Top 0.381: v81.39,99.81 v100.91,99.81 | v81.39,91.34 81.03,91.71 v24.68,91.71 | v24.68,120.8 v4.84,120.8
  Bottom 0.381: v100.91,99.81 100.91,105.33 B1.A8 | v81.39,91.34 v81.39,99.81 | v24.68,120.8 v24.68,91.71 | v4.84,120.8 4.84,122.28 P2.C
PORTK1  (via drill 0.35)
  Top 0.381: v74.4,107.54 94.65,107.54 95.39,108.28 100.91,108.28 103.49,105.7 B1.A9 | v38.3,110.49 v70.34,110.49 | v9.99,123.75 v33.88,123.75
  Bottom 0.381: v74.4,107.54 70.34,107.54 v70.34,110.49 | v38.3,110.49 34.99,113.81 34.99,122.64 v33.88,123.75 | v9.99,123.75 9.63,123.38 9.63,121.17 7.42,118.96 4.84,118.96 P2.D
PORTK2  (via drill 0.35)
  Top 0.381: v72.19,113.81 97.6,113.81 105.7,105.7 B1.A10 | v38.3,111.96 v70.34,111.96 | v32.78,120.07 33.88,118.96 33.88,117.12 5.21,117.12 v4.84,116.75
  Bottom 0.381: v70.34,111.96 v72.19,113.81 | v38.3,111.96 35.73,114.54 35.73,123.38 34.25,124.85 32.78,124.85 v32.78,120.07 | v4.84,116.75 4.84,114.91 P2.E
PORTK3  (via drill 0.35)
  Top 0.381: v71.08,114.91 99.07,114.91 108.28,105.7 B1.A11 | v38.3,113.44 v68.87,113.44 | v9.63,116.01 v31.67,116.01
  Bottom 0.381: v71.08,114.91 69.61,113.44 v68.87,113.44 | v38.3,113.44 36.46,115.28 36.46,123.75 34.62,125.59 31.67,125.59 v31.67,116.01 | v9.63,116.01 9.63,113.44 7.05,110.86 4.84,110.86 P2.F
PORTK4  (via drill 0.35)
  Top 0.381: v69.98,116.01 100.55,116.01 110.86,105.7 B1.A12 | v38.67,114.54 v67.77,114.54 | v33.88,126.69 32.78,125.59 v11.1,125.59
  Bottom 0.381: v69.98,116.01 68.5,114.54 v67.77,114.54 | v38.67,114.54 37.2,116.01 37.2,124.12 34.62,126.69 v33.88,126.69 | v11.1,125.59 11.1,110.86 7.05,106.81 4.84,106.81 P2.H
PORTK5  (via drill 0.35)
  Top 0.381: v68.14,117.86 101.28,117.86 113.44,105.7 B1.A13 | v38.3,117.86 v64.45,117.86 | v33.52,128.91 31.3,126.69 v12.94,126.69
  Bottom 0.381: v64.45,117.86 v68.14,117.86 | v38.3,117.86 37.94,118.22 37.94,125.59 34.62,128.91 v33.52,128.91 | v12.94,126.69 12.21,125.96 12.21,107.91 7.42,103.12 4.84,103.12 P2.J
PORTK6  (via drill 0.35)
  Top 0.381: v111.23,102.76 113.44,102.76 116.01,105.33 B1.A14 | v111.23,69.24 45.3,69.24 44.56,69.98 v14.41,69.98 | v4.84,96.86 v14.41,96.86
  Bottom 0.381: v111.23,69.24 v111.23,102.76 | v14.41,96.86 v14.41,69.98 | v4.84,96.86 4.84,98.7 P2.K
PORTK7  (via drill 0.35)
  Top 0.381: v118.59,89.5 92.81,89.5 88.76,85.45 48.25,85.45 43.83,89.86 23.94,89.86 21.73,92.08 21.73,103.86 v9.99,103.86
  Bottom 0.381: v118.59,89.5 118.59,105.33 B1.A15 | v9.99,103.86 9.63,103.49 9.63,97.6 7.05,95.02 4.84,95.02 P2.L
PROCESSOROVERRIDE  (via drill 0.35)
  Top 0.381: v88.76,96.86 89.13,96.5 127.06,96.5 v127.43,96.86 | v291.32,125.22 290.96,125.59 264.44,125.59 261.86,128.17 175.31,128.17 v173.84,126.69 | v173.1,128.91 125.96,128.91 124.12,130.75 B1.39
  Bottom 0.381: v88.76,96.86 85.08,93.18 85.08,81.39 82.13,78.45 1C.2 | v127.43,96.86 127.43,127.43 124.12,130.75 B1.39 | v291.32,125.22 291.32,117.12 293.9,117.12 296.11,114.91 P1.5 | v173.84,126.69 173.1,127.43 v173.1,128.91
PROCESSORREADY  (via drill 0.35)
  Top 0.381: v85.81,71.82 93.18,71.82 99.44,78.08 2C.2 | v98.7,131.48 120.8,131.48 121.17,131.12 B1.38
  Bottom 0.381: v85.81,71.82 85.81,92.08 98.7,104.97 v98.7,131.48
RESETVRAMPC  (via drill 0.35)
  Top 0.381: v93.55,83.6 95.39,85.45 v201.09,85.45 | v205.14,125.96 215.82,125.96 216.93,124.85 229.08,124.85 229.45,125.22 246.02,125.22 248.6,122.64 260.76,122.64 265.91,117.49 291.32,117.49 293.9,114.91 296.11,114.91 P1.E
  Bottom 0.381: v93.55,83.6 93.55,54.14 89.86,50.46 1D.12 | v201.09,85.45 201.09,103.12 205.14,107.17 v205.14,125.96
VCC
  Top 1.016: 127.64,94.61 127.64,87 C4.1 | C3.1 88.27,94.61
  Top 2.032: P2.A 4.83,128.91 P2.B | P1.1 296.16,128.91 P1.2
  Top 2.54: 36.2,173.99 36.2,102.23 43.81,94.61 88.27,94.61 127.64,94.61 | X1.1 44.23,173.76 44.45,173.99
  Top 5.08: 4.83,128.91 10.16,128.91 13.97,132.72 13.97,173.99 36.2,173.99 44.45,173.99 287.02,173.99 287.02,132.72 290.83,128.91 296.16,128.91
  Bottom 1.016: 4A.16 164.47,151.76 | 164.47,173.99 164.47,151.76 | 5A.16 182.25,163.19 | 182.25,163.19 182.25,172.72 180.97,173.99 | 6A.24 210.19,163.19 | 210.19,173.99 210.19,163.19 | 7A.24 233.04,163.19 | 233.04,173.99 233.04,163.19 | 8A.20 253.37,160.66 | 253.37,173.99 253.37,160.66 | 9A.20 269.88,160.66 | 269.88,173.99 269.88,160.66 | 164.47,151.76 164.47,113.67 | 164.47,113.67 164.47,88.9 | 164.47,88.9 164.47,71.75 | 164.47,71.75 164.47,31.11 4E.16 | 4C.16 164.47,71.75 | 4B.16 164.47,113.67 | 182.25,163.19 182.25,123.83 | 182.25,123.83 182.25,88.9 | 182.25,88.9 182.25,81.92 | 182.25,81.92 182.25,41.27 5E.16 | 5C.16 182.25,81.92 | 5B.16 182.25,123.83 | 210.19,163.19 210.19,123.83 | 210.19,123.83 210.19,88.9 | 210.19,88.9 210.19,81.92 | 210.19,81.92 210.19,41.27 6E.24 | 6C.24 210.19,81.92 | 6B.24 210.19,123.83 | 233.04,163.19 233.04,123.83 | 233.04,123.83 233.04,88.9 | 233.04,88.9 233.04,81.92 | 233.04,81.92 233.04,41.27 7E.24 | 7C.24 233.04,81.92 | 7B.24 233.04,123.83 | 253.37,160.66 253.37,121.28 | 253.37,121.28 253.37,88.9 | 253.37,88.9 253.37,79.38 | 253.37,79.38 253.37,38.73 8E.20 | 269.88,160.66 269.88,121.28 | 269.88,121.28 269.88,88.9 | 269.88,88.9 269.88,79.38 | 269.88,79.38 269.88,38.73 9E.20 | C9.1 253.37,88.9 | C10.1 269.88,88.9 | C8.1 233.04,88.9 | C7.1 210.19,88.9 | C6.1 182.25,88.9 | C5.1 164.47,88.9 | 8C.20 253.37,79.38 | 9C.20 269.88,79.38 | 8B.20 253.37,121.28 | 9B.20 269.88,121.28 | C4.1 127.64,87 127.64,81.92 | 127.64,81.92 3C.16 | 127.64,81.92 127.64,56.52 | 127.64,56.52 127.64,31.11 3E.16 | 3D.16 127.64,56.52 | 109.86,55.24 109.86,31.11 2E.16 | 109.86,80.64 109.86,55.24 | 109.86,80.64 109.86,87 92.08,87 | 109.86,80.64 2C.14 | 92.08,87 C3.1 | 2D.14 109.86,55.24
  Bottom 1.016: 109.86,55.24 R3.1 | 1D.14 92.08,55.24 92.08,80.64 | 92.08,80.64 92.08,87 | 1C.14 92.08,80.64
  Bottom 2.032: P2.B 4.83,128.91 P2.A | P1.1 296.16,128.91 P1.2
  Bottom 2.54: X1.1 44.23,173.76 44.45,173.99
  Bottom 5.08: 4.83,128.91 10.16,128.91 13.97,132.72 13.97,173.99 44.45,173.99 164.47,173.99 180.97,173.99 210.19,173.99 233.04,173.99 253.37,173.99 269.88,173.99 287.02,173.99 287.02,132.72 290.83,128.91 296.16,128.91
VPC0  (via drill 0.35)
  Top 0.381: v159.84,33.15 132.22,33.15 125.22,26.15 3E.14
  Bottom 0.381: 4E.10 161.68,16.2 159.84,18.05 v159.84,33.15 158.74,34.25 158.74,39.41 159.11,39.78 159.11,95.76 161.68,98.34 4B.10
VPC1  (via drill 0.35)
  Top 0.381: v158.74,32.04 158.37,32.41 134.06,32.41 125.22,23.57 3E.13 | v158.74,23.57 161.68,23.57 4E.13
  Bottom 0.381: v158.74,23.57 v158.74,32.04 158,32.78 158,39.78 158.37,40.15 158.37,102.39 161.68,105.7 4B.13
VPC2  (via drill 0.35)
  Top 0.381: 3E.12 125.22,20.99 134.06,29.83 v145.85,29.83 170.89,29.83 172,28.73 5E.6 | v145.85,115.65 165.37,115.65 169.42,111.59 171.63,111.59 172,111.23 5B.6
  Bottom 0.381: v145.85,29.83 v145.85,115.65
VPC3  (via drill 0.35)
  Top 0.381: v174.21,44.56 v148.06,44.56 v128.91,44.56 | v147.69,118.59 172,118.59 5B.3
  Bottom 0.381: v128.91,44.56 128.91,22.1 125.22,18.41 3E.11 | v174.21,44.56 174.21,38.3 172.36,36.46 5E.3 | v147.69,118.59 147.69,65.56 148.06,65.19 v148.06,44.56
VPC4
  Top 0.381: 3D.14 132.59,58.93 153.95,58.93 4C.6
  Bottom 0.381: 4A.6 154.32,138.85 155.42,137.74 157.63,137.74 157.63,62.24 154.32,58.93 4C.6
VPC5  (via drill 0.35)
  Top 0.381: v178.26,62.61 177.52,63.35 177.52,65.93 178.62,65.93 179.36,66.66 5C.10 | 3D.13 125.22,48.98 126.69,50.46 v178.26,50.46 v185.99,50.46 | v178.99,144 177.52,144 177.52,145.85 179.36,147.69 5A.10 | v178.99,126.33 185.62,126.33 v185.99,125.96
  Bottom 0.381: v178.26,62.61 v178.26,50.46 | v178.99,126.33 v178.99,144 | v185.99,50.46 v185.99,125.96
VPC6  (via drill 0.35)
  Top 0.381: v177.52,46.04 v138.11,46.04 125.22,46.04 3D.12 | v162.42,153.21 163.16,153.21 164.63,151.74 173.47,151.74 174.57,152.84 176.78,152.84 179.36,155.42 5A.13 | v160.95,155.79 158.37,153.21 149.53,153.21 v138.11,141.8
  Bottom 0.381: v177.52,46.04 177.15,46.41 177.15,71.82 179.36,74.03 5C.13 | v162.42,153.21 160.95,154.69 v160.95,155.79 | v138.11,46.04 v138.11,141.8
VPC7  (via drill 0.35)
  Top 0.381: v143.64,43.46 125.22,43.46 3D.11 | v143.64,76.24 144,76.61 172,76.61 5C.3 | v142.53,120.43 v165.74,120.43
  Bottom 0.381: v143.64,43.46 v143.64,76.24 142.53,77.34 v142.53,120.43 | v165.74,120.43 165.74,155.42 169.42,155.42 172,158 5A.3
VPC8  (via drill 0.35)
  Top 0.381: v163.16,78.82 143.64,78.82 142.16,77.34 v133.69,77.34 125.59,77.34 125.22,76.97 3C.14 | v163.16,73.29 167.21,69.24 172,69.24 5C.6 | v167.94,119.7 167.58,119.33 148.43,119.33 148.06,119.7 143.27,119.7 142.9,119.33 v133.69,119.33
  Bottom 0.381: v163.16,73.29 v163.16,78.82 | v167.94,119.7 167.94,146.22 172,150.27 5A.6 | v133.69,77.34 v133.69,119.33
VPC9  (via drill 0.35)
  Top 0.381: v160.21,79.92 159.84,79.55 v135.9,79.55 127.8,79.55 126.33,78.08 123.75,78.08 123.01,77.34 123.01,74.4 124.85,74.4 3C.13
  Bottom 0.381: v160.21,79.92 159.84,79.55 159.84,66.29 161.68,64.45 4C.13 | v135.9,79.55 135.9,97.6 137.01,98.7 137.01,142.9 156.9,142.9 157.63,143.64 157.63,144 161.68,144 4A.13
VPC10  (via drill 0.35)
  Top 0.381: v166.84,77.71 143.64,77.71 142.16,76.24 129.64,76.24 125.22,71.82 3C.12 | v166.84,22.1 175.68,22.1 179.36,25.78 5E.10 | v166.84,94.65 v177.52,94.65
  Bottom 0.381: v166.84,22.1 v166.84,77.71 v166.84,94.65 | v177.52,94.65 177.52,106.44 179.36,108.28 5B.10
VPC11  (via drill 0.35)
  Top 0.381: v156.53,74.4 144.74,74.4 | 144.74,74.4 130.38,74.4 125.22,69.24 3C.11 | v144.74,18.41 4E.6 | 144.74,74.4 v144.74,74.03
  Bottom 0.381: v156.53,74.4 156.9,74.77 156.9,98.34 154.32,100.91 4B.6 | v144.74,74.03 v144.74,18.41
VRAM0  (via drill 0.35)
  Top 0.381: v276.96,33.88 267.39,33.88 9E.18 | v276.96,85.08 276.59,85.45 273.65,85.45 272.91,86.18 272.91,89.13 274.38,89.13 276.59,91.34 276.59,97.6 275.86,98.34 v274.38,98.34 | v274.38,116.01 267.39,116.01 9B.18 | v280.64,90.97 296.11,90.97 P1.M
  Bottom 0.381: v276.96,85.08 v276.96,33.88 | v274.38,116.01 v274.38,98.34 274.38,96.86 279.54,91.71 279.91,91.71 v280.64,90.97
VRAM1  (via drill 0.35)
  Top 0.381: v255.6,27.25 265.91,27.25 267.02,28.36 9E.16 | v255.6,114.91 263.33,114.91 267.02,111.23 9B.16 267.39,110.86 v273.28,110.86 | v280.64,89.5 281.01,89.13 293.9,89.13 296.11,86.92 P1.N
  Bottom 0.381: v255.6,27.25 255.97,27.62 255.97,114.54 v255.6,114.91 | v280.64,89.5 273.28,96.86 v273.28,110.86
VRAM2  (via drill 0.35)
  Top 0.381: v282.49,23.57 267.39,23.57 9E.14 | v286.91,82.87 296.11,82.87 P1.P | v286.91,105.7 267.39,105.7 9B.14
  Bottom 0.381: v282.49,23.57 282.49,69.98 286.91,74.4 v286.91,82.87 v286.91,105.7
VRAM3  (via drill 0.35)
  Top 0.381: v272.17,100.91 267.39,100.91 9B.12 | v282.49,79.18 296.11,79.18 P1.R
  Bottom 0.381: 272.54,87.66 272.54,100.55 v272.17,100.91 | 272.54,87.66 272.54,23.57 267.39,18.41 9E.12 | v282.49,79.18 282.49,83.6 278.44,87.66 272.54,87.66
VRAM4  (via drill 0.35)
  Top 0.381: v280.28,20.99 267.39,20.99 9E.13 | v281.38,75.87 295.38,75.87 296.11,75.13 P1.S | v278.44,85.08 278.8,85.08 278.8,96.5 273.28,102.02 268.86,102.02 267.39,103.49 9B.13
  Bottom 0.381: 280.28,74.77 v280.28,20.99 | v281.38,75.87 280.28,74.77 | v278.44,85.08 280.28,83.24 280.28,74.77
VRAM5  (via drill 0.35)
  Top 0.381: v279.17,26.15 267.39,26.15 9E.15 | v279.17,69.61 280.28,70.71 v288.01,70.71 296.11,70.71 P1.T | v288.01,108.28 267.39,108.28 9B.15
  Bottom 0.381: v279.17,69.61 v279.17,26.15 | v288.01,70.71 v288.01,108.28
VRAM6  (via drill 0.35)
  Top 0.381: v283.59,31.3 267.39,31.3 9E.17 | P1.U 296.11,67.03 v283.59,67.03 v281.38,67.03 | v284.7,112.33 268.49,112.33 267.39,113.44 9B.17
  Bottom 0.381: v283.59,67.03 v283.59,31.3 | v284.7,112.33 284.7,73.29 281.38,69.98 v281.38,67.03
VRAM7  (via drill 0.35)
  Top 0.381: v265.18,57.82 v273.65,57.82 279.91,57.82 284.33,62.24 295.38,62.24 296.11,62.98 P1.V | v277.7,118.59 267.39,118.59 9B.19 | v277.7,96.13 277.7,86.55 v274.01,86.55
  Bottom 0.381: v265.18,57.82 265.18,38.3 267.02,36.46 9E.19 | v277.7,96.13 v277.7,118.59 | v274.01,86.55 273.65,86.18 v273.65,57.82
VRAM8  (via drill 0.35)
  Top 0.381: v296.11,92.81 v279.91,92.81 279.54,92.81 279.54,83.6 271.81,75.87 268.86,75.87 267.39,74.4 9C.18 | v276.59,155.42 267.39,155.42 9A.18
  Bottom 0.381: v296.11,92.81 296.11,90.97 P1.11 | v276.59,155.42 276.59,95.76 279.54,92.81 v279.91,92.81
VRAM9  (via drill 0.35)
  Top 0.381: v296.11,84.71 280.28,84.71 280.28,74.77 276.23,70.71 268.86,70.71 267.39,69.24 9C.16 | v290.22,123.38 v261.49,123.38
  Bottom 0.381: 296.11,86.92 v296.11,84.71 | v261.49,123.38 261.49,126.33 262.6,127.43 262.6,145.85 267.02,150.27 9A.16 | v290.22,123.38 290.59,123.01 290.59,90.6 294.27,86.92 296.11,86.92 | 296.11,86.92 P1.12
VRAM10  (via drill 0.35)
  Top 0.381: v288.75,68.14 277.33,68.14 274.38,65.19 268.12,65.19 267.39,64.45 9C.14 | v288.38,126.69 286.91,126.69 269.23,144.37 268.12,144.37 267.39,145.11 9A.14
  Bottom 0.381: v288.75,68.14 289.12,68.5 289.12,78.08 | 289.12,78.08 293.9,82.87 296.11,82.87 P1.13 | v288.38,126.69 289.12,125.96 289.12,78.08
VRAM11  (via drill 0.35)
  Top 0.381: v264.81,62.61 264.81,61.51 267.02,59.3 9C.12 267.39,59.3 v274.75,59.3 | v281.38,81.03 v296.11,81.03
  Bottom 0.381: v264.81,62.61 264.44,62.98 264.44,137.74 267.02,140.32 9A.12 | v296.11,81.03 296.11,79.18 P1.14 | v281.38,81.03 281.01,81.39 281.01,83.97 278.8,86.18 275.12,86.18 275.12,72.56 274.75,72.19 v274.75,59.3
VRAM12  (via drill 0.35)
  Top 0.381: v289.85,63.35 284.33,63.35 283.59,62.61 268.12,62.61 267.39,61.87 9C.13
  Bottom 0.381: v289.85,63.35 289.85,72.92 291.69,74.77 296.11,74.77 P1.15 | 9A.13 267.02,142.53 263.7,139.22 263.7,62.24 264.44,61.51 267.02,61.51 9C.13
VRAM13  (via drill 0.35)
  Top 0.381: v296.11,73.29 291.69,73.29 290.22,74.77 v285.8,74.77 282.85,74.77 275.86,67.77 268.12,67.77 267.39,67.03 9C.15 | v284.7,130.38 284.33,130.38 284.33,131.12 268.49,146.95 268.12,146.95 267.39,147.69 9A.15
  Bottom 0.381: v296.11,73.29 296.11,71.08 P1.16 | v284.7,130.38 285.8,129.27 v285.8,74.77
VRAM14  (via drill 0.35)
  Top 0.381: v275.86,71.82 267.39,71.82 9C.17 267.02,71.82 265.18,71.82 265.18,82.5 274.01,91.34 275.49,91.34 v275.49,97.23 | v296.11,65.19 v275.86,65.19 | v275.49,152.84 267.39,152.84 9A.17
  Bottom 0.381: v275.86,65.19 v275.86,71.82 | v296.11,65.19 296.11,67.03 P1.17 | v275.49,97.23 v275.49,152.84
VRAM15  (via drill 0.35)
  Top 0.381: v271.44,76.97 267.39,76.97 9C.19 | v271.44,158 267.39,158 9A.19 | v296.11,61.14 295.75,60.77 283.96,60.77 279.91,56.72 v271.44,56.72
  Bottom 0.381: v271.44,158 271.07,157.63 271.07,77.34 v271.44,76.97 v271.44,56.72 | v296.11,61.14 296.11,62.98 P1.18
VRAM_A_0
  Top 0.508: 6B.9 205.19,103.5 206.46,104.78 208.83,104.78 210.1,103.5 7B.9 215.67,103.91 216.81,103.91 217.67,104.78 231.78,104.78 241.94,114.94 244.47,114.94 245.75,116.2 8B.18 9B.3
VRAM_A_1
  Top 0.508: 6B.10 205.19,100.97 206.46,102.23 208.83,102.23 210.1,100.97 7B.10 215.67,101.37 216.81,101.37 217.67,102.23 234.4,102.23 242.02,109.86 244.47,109.86 245.75,111.12 8B.16 9B.5
VRAM_A_2
  Top 0.508: 6B.11 205.19,98.42 206.46,99.69 208.83,99.69 210.1,98.42 7B.11 215.67,98.83 216.81,98.83 217.67,99.69 236.94,99.69 242.02,104.78 244.47,104.78 245.75,106.05 8B.14 9B.7
VRAM_A_3
  Top 0.508: 6B.13 212.81,95.89 214.08,94.61 216.45,94.61 217.72,95.89 7B.13 238.12,95.89 241.94,99.69 244.39,99.69 245.66,100.97 8B.12 9B.9
VRAM_A_4
  Top 0.508: 6B.14 208.88,98.42 210.15,97.16 216.45,97.16 217.72,98.42 7B.14 238.21,98.42 242.02,102.23 244.47,102.23 245.75,103.5 8B.13 9B.8
VRAM_A_5
  Top 0.508: 6B.15 208.88,100.97 210.15,99.69 216.45,99.69 217.72,100.97 7B.15 235.67,100.97 242.02,107.31 244.47,107.31 245.75,108.58 8B.15 9B.6
VRAM_A_6
  Top 0.508: 6B.16 208.88,103.5 210.15,102.23 216.45,102.23 217.72,103.5 7B.16 233.04,103.5 241.94,112.39 244.39,112.39 245.66,113.67 8B.17 9B.4
VRAM_A_7
  Top 0.508: 6B.17 208.88,106.05 210.15,104.78 216.45,104.78 217.72,106.05 7B.17 241.94,117.47 244.47,117.47 245.75,118.75 8B.19 9B.2
VRAM_A_8
  Top 0.508: 6A.9 205.19,142.88 206.46,144.15 208.83,144.15 210.1,142.88 7A.9 215.67,143.28 217.44,143.28 218.31,144.15 231.78,144.15 241.94,154.31 244.39,154.31 245.66,155.57 8A.18 9A.3
VRAM_A_9
  Top 0.508: 6A.10 205.19,140.34 206.46,141.6 208.83,141.6 210.1,140.34 7A.10 215.67,140.74 217.44,140.74 218.31,141.6 234.4,141.6 242.02,149.22 244.47,149.22 245.75,150.5 8A.16 9A.5
VRAM_A_10
  Top 0.508: 6A.11 205.19,137.79 206.46,139.06 208.83,139.06 210.1,137.79 7A.11 215.67,138.2 217.44,138.2 218.31,139.06 236.85,139.06 241.94,144.15 244.39,144.15 245.66,145.41 8A.14 9A.7
VRAM_A_11
  Top 0.508: 6A.13 212.81,135.25 214.08,133.99 217.09,133.99 218.36,135.25 7A.13 238.12,135.25 241.94,139.06 244.39,139.06 245.66,140.34 8A.12 9A.9
VRAM_A_12
  Top 0.508: 6A.14 208.88,137.79 210.15,136.53 217.09,136.53 218.36,137.79 7A.14 238.12,137.79 241.94,141.6 244.39,141.6 245.66,142.88 8A.13 9A.8
VRAM_A_13
  Top 0.508: 6A.15 208.88,140.34 210.15,139.06 217.09,139.06 218.36,140.34 7A.15 235.59,140.34 241.94,146.69 244.39,146.69 245.66,147.96 8A.15 9A.6
VRAM_A_14
  Top 0.508: 6A.16 208.88,142.88 210.15,141.6 217.09,141.6 218.36,142.88 7A.16 233.13,142.88 242.02,151.76 244.47,151.76 245.75,153.03 8A.17 9A.4
VRAM_A_15
  Top 0.508: 6A.17 208.88,145.41 210.15,144.15 217.09,144.15 218.36,145.41 7A.17 241.94,156.84 244.39,156.84 245.66,158.12 8A.19 9A.2
VRAM_B_0
  Top 0.508: 6E.9 205.19,20.95 206.46,22.23 208.83,22.23 210.1,20.95 7E.9 215.67,21.36 216.81,21.36 217.67,22.23 231.86,22.23 242.02,32.38 244.47,32.38 245.75,33.66 8E.18 9E.3
VRAM_B_1
  Top 0.508: 6E.10 205.19,18.41 206.46,19.68 208.83,19.68 210.1,18.41 7E.10 215.67,18.82 216.81,18.82 217.67,19.68 234.4,19.68 242.02,27.3 244.47,27.3 245.75,28.57 8E.16 9E.5
VRAM_B_2
  Top 0.508: 6E.11 205.19,15.88 206.46,17.14 208.83,17.14 210.1,15.88 7E.11 215.67,16.28 216.81,16.28 217.67,17.14 236.85,17.14 241.94,22.23 244.39,22.23 245.66,23.5 8E.14 9E.7
VRAM_B_3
